ORGANIZATION_BLOCK OB 100
TITLE = "Complete Restart"
AUTHOR : Esposito
FAMILY : EGAL_srl
VERSION : 0.1


VAR_TEMP
  OB100_EV_CLASS : BYTE ;	//16#13, Event class 1, Entering event state, Event logged in diagnostic buffer
  OB100_STRTUP : BYTE ;	//16#81/82/83/84 Method of startup
  OB100_PRIORITY : BYTE ;	//27 (Priority of 1 is lowest)
  OB100_OB_NUMBR : BYTE ;	//100 (Organization block 100, OB100)
  OB100_RESERVED_1 : BYTE ;	//Reserved for system
  OB100_RESERVED_2 : BYTE ;	//Reserved for system
  OB100_STOP : WORD ;	//Event that caused CPU to stop (16#4xxx)
  OB100_STRT_INFO : DWORD ;	//Information on how system started
  OB100_DATE_TIME : DATE_AND_TIME ;	//Date and time OB100 started
  CONV_RET_VAL : INT ;
  CONV_RETURN_DB : WORD ;
END_VAR
BEGIN
NETWORK
TITLE =CALL SFC22 FOR CREATE THE DB11

      CALL SFC   22 (
           LOW_LIMIT                := W#16#B,
           UP_LIMIT                 := W#16#B,
           COUNT                    := W#16#800,
           RET_VAL                  := #CONV_RET_VAL,
           DB_NUMBER                := #CONV_RETURN_DB);

END_ORGANIZATION_BLOCK

